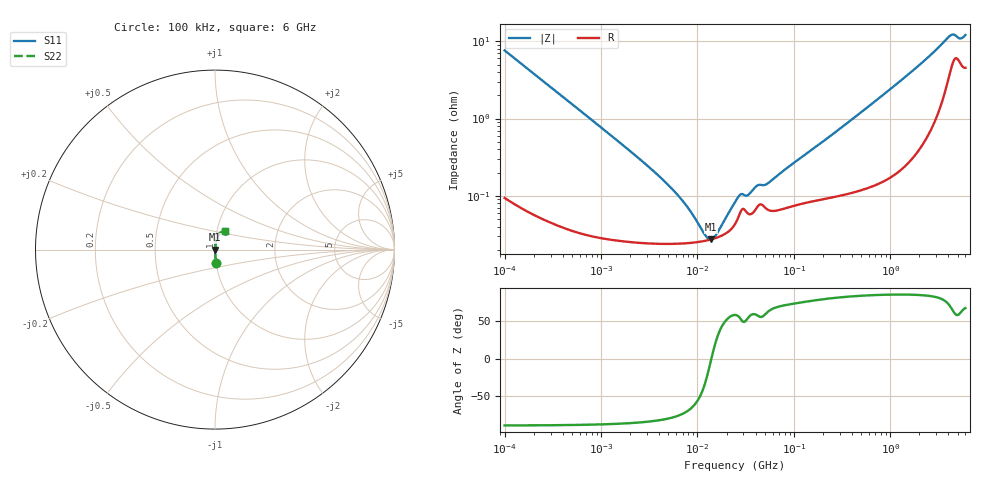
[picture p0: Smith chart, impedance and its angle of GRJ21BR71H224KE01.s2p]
!Murata Part Number: GRJ21BR71H224KE01
!These Parameters are Measured in Series Mode Connection
!Data Generated on Jun 19, 2026
!  o--ll--o
!Port1  Port2
!  o------o
!Operation Temp=25[degC], DC Bias Voltage=0[V]
!Freq. Start=100[kHz] Stop=6[GHz] 401[Steps]
# Hz S RI R 50
!Freq.(Hz) S11(Real) S11(Imag) S21(Real) S21(Imag) S12(Real) S12(Imag) S22(Real) S22(Imag)
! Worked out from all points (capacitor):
!   401 points, 100 kHz to 6 GHz, reference 50 ohm
!   read as one part in series: C = 209 nF near 105.7 kHz
!   lowest |Z| = 27.3 mohm at 13.75 MHz (marker M1)
!   series resonance near 13.93 MHz, so ESL is about 630 pH
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100000  0.00669 -0.0756  0.9933 0.0756  0.9933 0.0756  0.00669 -0.0756
631452  0.00047 -0.0122  0.9995 0.0122  0.9995 0.0122  0.00047 -0.0122
2060590  0.000265 -0.00367  0.9997 0.00367  0.9997 0.00367  0.000265 -0.00367
3987316  0.000243 -0.00179  0.9998 0.00179  0.9998 0.00179  0.000243 -0.00179
6911753  0.000242 -0.000848  0.9998 0.000848  0.9998 0.000848  0.000242 -0.000848
8853126  0.000248 -0.000524  0.9998 0.000524  0.9998 0.000524  0.000248 -0.000524
1.198108e7  0.000262 -0.00017  0.9997 0.00017  0.9997 0.00017  0.000262 -0.00017
1.301164e7  0.000268 -7.66e-05  0.9997 7.66e-05  0.9997 7.66e-05  0.000268 -7.66e-05
1.374747e7  0.000272 -1.48e-05  0.9997 1.48e-05  0.9997 1.48e-05  0.000272 -1.48e-05
1.577428e7  0.000287 0.000141  0.9997 -0.000141  0.9997 -0.000141  0.000287 0.000141
2.517799e7  0.000458 0.000747  0.9995 -0.000747  0.9995 -0.000747  0.000458 0.000747
2.810622e7  0.000629 0.000837  0.9994 -0.000837  0.9994 -0.000837  0.000629 0.000837
3.407377e7  0.000581 0.000866  0.9994 -0.000866  0.9994 -0.000866  0.000581 0.000866
4.246031e7  0.00074 0.00116  0.9993 -0.00116  0.9993 -0.00116  0.00074 0.00116
5.438656e7  0.000657 0.00131  0.9993 -0.00131  0.9993 -0.00131  0.000657 0.00131
1.546735e8  0.00086 0.00388  0.9991 -0.00388  0.9991 -0.00388  0.00086 0.00388
9.76689e8  0.00224 0.0234  0.9978 -0.0234  0.9978 -0.0234  0.00224 0.0234
2.702311e9  0.0122 0.0673  0.9878 -0.0673  0.9878 -0.0673  0.0122 0.0673
4.082404e9  0.0456 0.1014  0.9544 -0.1014  0.9544 -0.1014  0.0456 0.1014
4.433555e9  0.0599 0.0991  0.9401 -0.0991  0.9401 -0.0991  0.0599 0.0991
5.374892e9  0.0561 0.0864  0.9439 -0.0864  0.9439 -0.0864  0.0561 0.0864
6e9  0.0543 0.1012  0.9457 -0.1012  0.9457 -0.1012  0.0543 0.1012
